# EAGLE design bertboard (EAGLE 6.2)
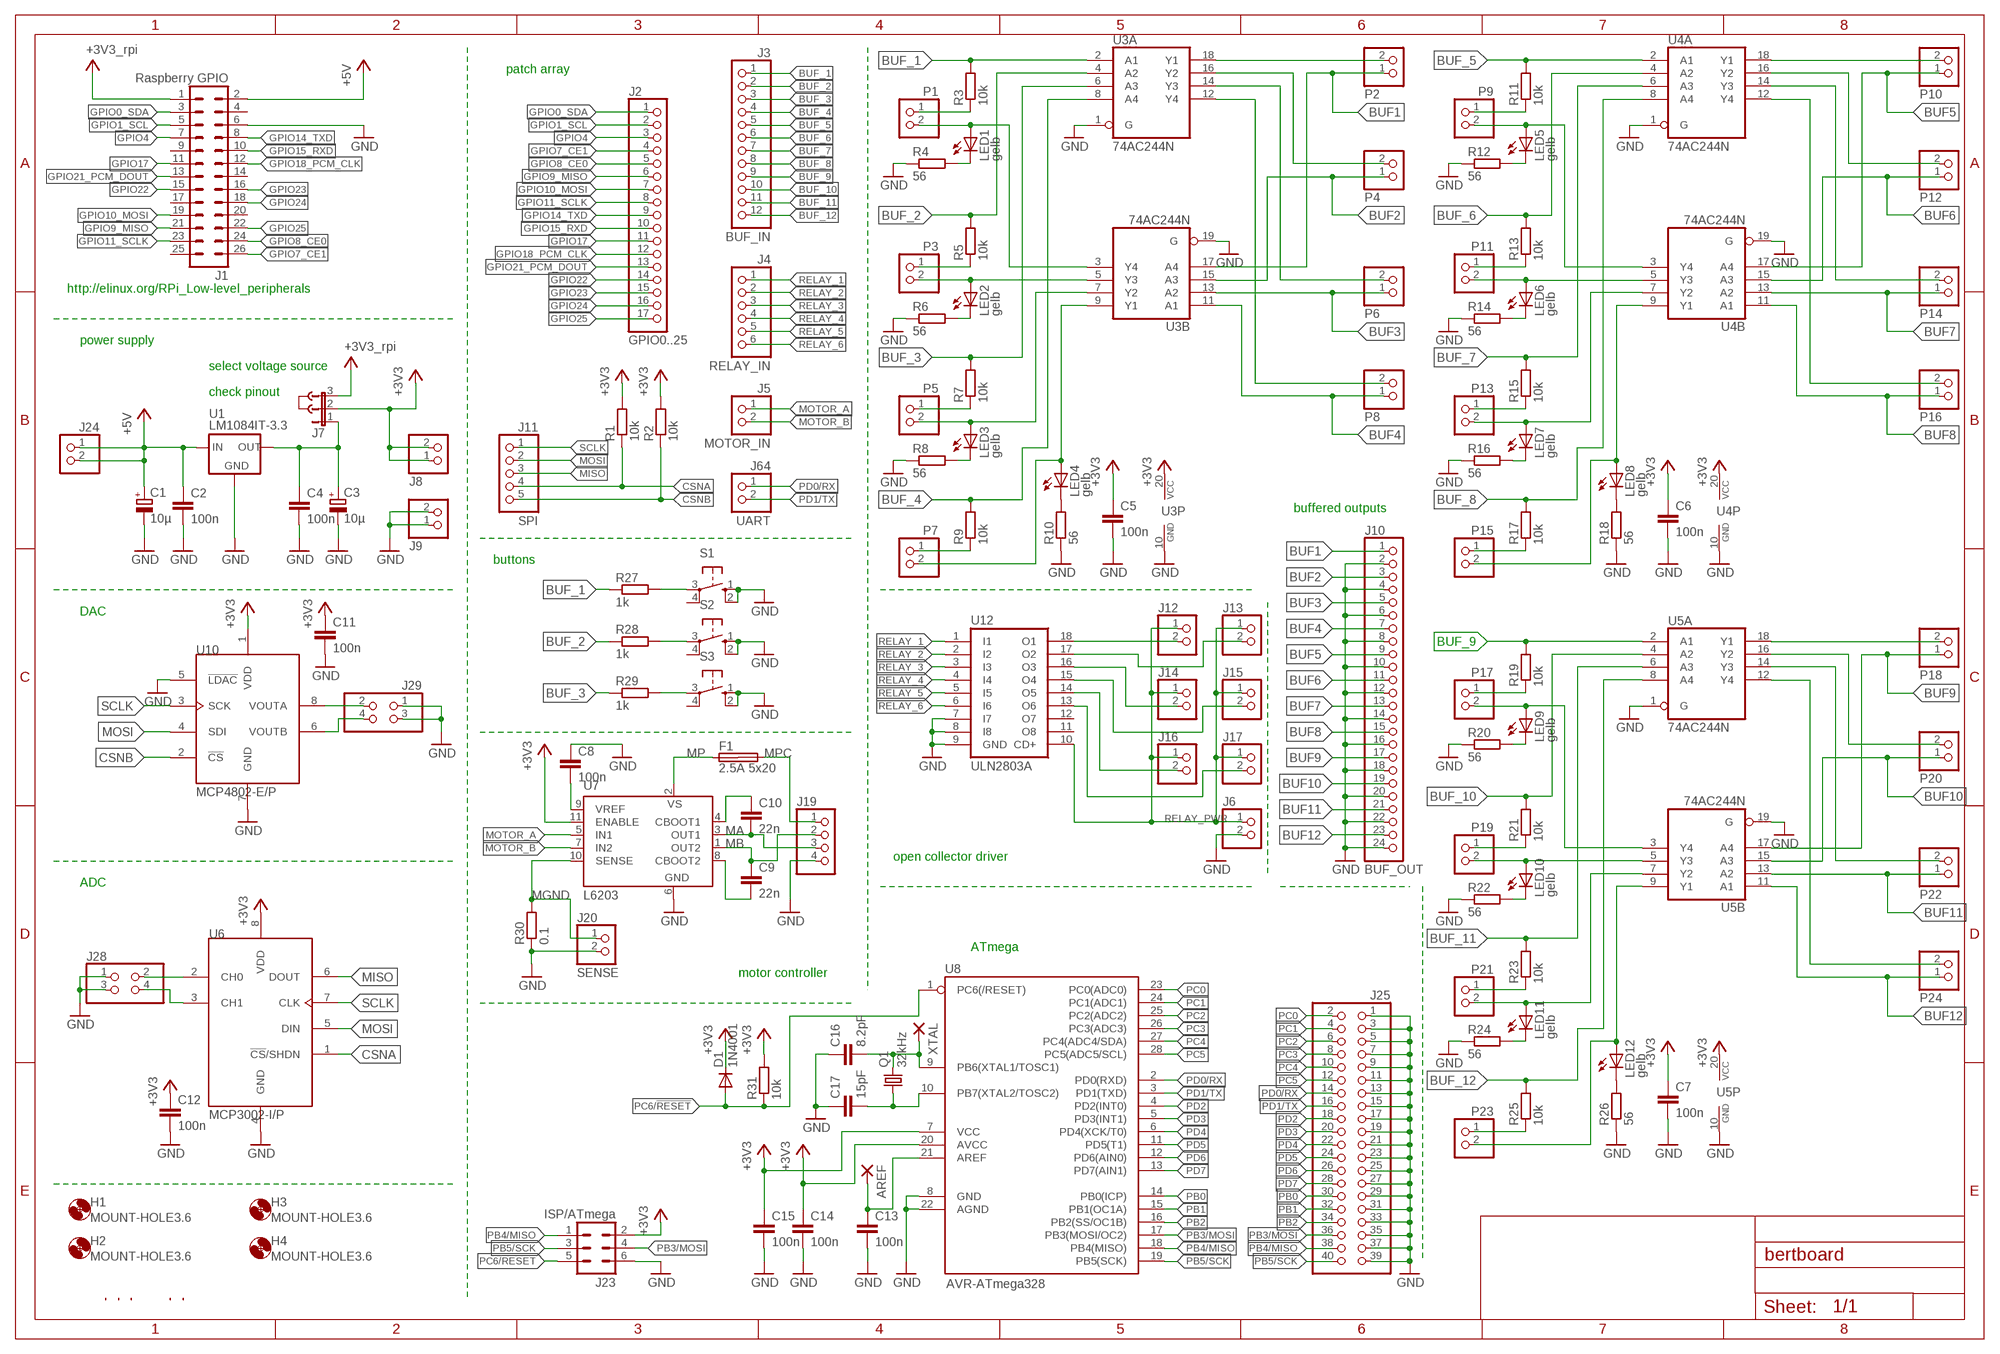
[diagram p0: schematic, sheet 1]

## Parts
AREF  1,6/0,9  [1,6/0,9]
C1  10µ  CPOL-EUE2-5  [E2-5]
C2  100n  C-EUC2012  [C2012]
C3  10µ  CPOL-EUE2-5  [E2-5]
C4  100n  C-EUC2012  [C2012]
C5  100n  C-EUC2012  [C2012]
C6  100n  C-EUC2012  [C2012]
C7  100n  C-EUC2012  [C2012]
C8  100n  C-EUC2012  [C2012]
C9  22n  C-EUC2012  [C2012]
C10  22n  C-EUC2012  [C2012]
C11  100n  C-EUC2012  [C2012]
C12  100n  C-EUC2012  [C2012]
C13  100n  C-EUC2012  [C2012]
C14  100n  C-EUC2012  [C2012]
C15  100n  C-EUC2012  [C2012]
C16  8.2pF  C-EUC2012  [C2012]
C17  15pF  C-EUC2012  [C2012]
D1  1N4001  1N4004  [DO41-10]
F1  2.5A 5x20  SHK20Q  [SHK20Q]
H1  MOUNT-HOLE3.6  [3,6]
H2  MOUNT-HOLE3.6  [3,6]
H3  MOUNT-HOLE3.6  [3,6]
H4  MOUNT-HOLE3.6  [3,6]
J1  Raspberry GPIO  ML26  [ML26]
J2  GPIO0..25  PINHD-1X17  [1X17]
J3  BUF_IN  PINHD-1X12  [1X12]
J4  RELAY_IN  PINHD-1X6  [1X06]
J5  MOTOR_IN  PINHD-1X2  [1X02]
J6  PINHD-1X2  [1X02]
J7  JP2E  [JP2]
J8  PINHD-1X2  [1X02]
J9  PINHD-1X2  [1X02]
J10  BUF_OUT  PINHD-1X24  [1X24]
J11  SPI  PINHD-1X5  [1X05]
J12  PINHD-1X2  [1X02]
J13  PINHD-1X2  [1X02]
J14  PINHD-1X2  [1X02]
J15  PINHD-1X2  [1X02]
J16  PINHD-1X2  [1X02]
J17  PINHD-1X2  [1X02]
J19  PINHD-1X4  [1X04]
J20  SENSE  PINHD-1X2  [1X02]
J23  ISP/ATmega  ML6  [ML6]
J24  PINHD-1X2  [1X02]
J25  PINHD-2X20  [2X20]
J28  PINHD-2X2  [2X02]
J29  PINHD-2X2  [2X02]
J64  UART  PINHD-1X2  [1X02]
J999  JUMPER  [JUMP]
LED1  gelb  LED3MM  [LED3MM]
LED2  gelb  LED3MM  [LED3MM]
LED3  gelb  LED3MM  [LED3MM]
LED4  gelb  LED3MM  [LED3MM]
LED5  gelb  LED3MM  [LED3MM]
LED6  gelb  LED3MM  [LED3MM]
LED7  gelb  LED3MM  [LED3MM]
LED8  gelb  LED3MM  [LED3MM]
LED9  gelb  LED3MM  [LED3MM]
LED10  gelb  LED3MM  [LED3MM]
LED11  gelb  LED3MM  [LED3MM]
LED12  gelb  LED3MM  [LED3MM]
P1  PINHD-1X2  [1X02]
P2  PINHD-1X2  [1X02]
P3  PINHD-1X2  [1X02]
P4  PINHD-1X2  [1X02]
P5  PINHD-1X2  [1X02]
P6  PINHD-1X2  [1X02]
P7  PINHD-1X2  [1X02]
P8  PINHD-1X2  [1X02]
P9  PINHD-1X2  [1X02]
P10  PINHD-1X2  [1X02]
P11  PINHD-1X2  [1X02]
P12  PINHD-1X2  [1X02]
P13  PINHD-1X2  [1X02]
P14  PINHD-1X2  [1X02]
P15  PINHD-1X2  [1X02]
P16  PINHD-1X2  [1X02]
P17  PINHD-1X2  [1X02]
P18  PINHD-1X2  [1X02]
P19  PINHD-1X2  [1X02]
P20  PINHD-1X2  [1X02]
P21  PINHD-1X2  [1X02]
P22  PINHD-1X2  [1X02]
P23  PINHD-1X2  [1X02]
P24  PINHD-1X2  [1X02]
Q1  32kHz  CRYSTALTC26H  [TC26H]
R1  10k  R-EU_M3216  [M3216]
R2  10k  R-EU_M3216  [M3216]
R3  10k  R-EU_M3216  [M3216]
R4  56  R-EU_M3216  [M3216]
R5  10k  R-EU_M3216  [M3216]
R6  56  R-EU_M3216  [M3216]
R7  10k  R-EU_M3216  [M3216]
R8  56  R-EU_M3216  [M3216]
R9  10k  R-EU_M3216  [M3216]
R10  56  R-EU_M3216  [M3216]
R11  10k  R-EU_M3216  [M3216]
R12  56  R-EU_M3216  [M3216]
R13  10k  R-EU_M3216  [M3216]
R14  56  R-EU_M3216  [M3216]
R15  10k  R-EU_M3216  [M3216]
R16  56  R-EU_M3216  [M3216]
R17  10k  R-EU_M3216  [M3216]
R18  56  R-EU_M3216  [M3216]
R19  10k  R-EU_M3216  [M3216]
R20  56  R-EU_M3216  [M3216]
R21  10k  R-EU_M3216  [M3216]
R22  56  R-EU_M3216  [M3216]
R23  10k  R-EU_M3216  [M3216]
R24  56  R-EU_M3216  [M3216]
R25  10k  R-EU_M3216  [M3216]
R26  56  R-EU_M3216  [M3216]
R27  1k  R-EU_M3216  [M3216]
R28  1k  R-EU_M3216  [M3216]
R29  1k  R-EU_M3216  [M3216]
R30  0.1  R-EU_R2512  [R2512]
R31  10k  R-EU_M3216  [M3216]
S1  10-XX  [B3F-10XX]
S2  10-XX  [B3F-10XX]
S3  10-XX  [B3F-10XX]
U1  LM1084IT-3.3  LM1084IT-XX  [LM1084IT-XX]
U3  74AC244N  [DIL20]
U4  74AC244N  [DIL20]
U5  74AC244N  [DIL20]
U6  MCP3002-I/P  [DIL-08]
U7  L6203  [MULTIWATT-11]
U8  AVR-ATmega328  AVR-MEGA8-PPTH  [DIL28-3]
U10  MCP4802-E/P  [DIL-08]
U12  ULN2803A  [DIL18]
U$1  MARKTRIANGLE  [MARK_TRIANGLE]
U$2  MARKTRIANGLE  [MARK_TRIANGLE]
U$3  MARKTRIANGLE  [MARK_TRIANGLE]
U$9  MARKGND  [MARK_GND]
U$19  MARKGND  [MARK_GND]
XTAL  1,6/0,9  [1,6/0,9]

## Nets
+3V3 [Power]: C5.1 C6.1 C7.1 C11.1 C12.1 C14.1 C15.1 D1.C J7.2 J8.1 J8.2 J23.2 R1.2 R2.2 R31.2 U3.20(P:VCC) U4.20(P:VCC) U5.20(P:VCC) U6.8(VDD) U7.11(ENABLE) U8.7(VCC) U8.20(AVCC) U10.1(VDD)
+5V [Power]: C1.+ C2.1 J1.2 J24.1 J24.2 U1.INPUT(IN)
AD0: J28.2 U6.2(CH0)
AD1: J28.4 U6.3(CH1)
BUF1: J10.1 P2.1 U3.17(B:A4)
BUF2: J10.3 P4.1 U3.15(B:A3)
BUF3: J10.5 P6.1 U3.13(B:A2)
BUF4: J10.7 P8.1 U3.11(B:A1)
BUF5: J10.9 P10.1 U4.17(B:A4)
BUF6: J10.11 P12.1 U4.15(B:A3)
BUF7: J10.13 P14.1 U4.13(B:A2)
BUF8: J10.15 P16.1 U4.11(B:A1)
BUF9: J10.17 P18.1 U5.17(B:A4)
BUF10: J10.19 P20.1 U5.15(B:A3)
BUF11: J10.21 P22.1 U5.13(B:A2)
BUF12: J10.23 P24.1 U5.11(B:A1)
BUF_1: J3.1 R3.2 R27.1 U3.2(A:A1)
BUF_2: J3.2 R5.2 R28.1 U3.4(A:A2)
BUF_3: J3.3 R7.2 R29.1 U3.6(A:A3)
BUF_4: J3.4 R9.2 U3.8(A:A4)
BUF_5: J3.5 R11.2 U4.2(A:A1)
BUF_6: J3.6 R13.2 U4.4(A:A2)
BUF_7: J3.7 R15.2 U4.6(A:A3)
BUF_8: J3.8 R17.2 U4.8(A:A4)
BUF_9: J3.9 R19.2 U5.2(A:A1)
BUF_10: J3.10 R21.2 U5.4(A:A2)
BUF_11: J3.11 R23.2 U5.6(A:A3)
BUF_12: J3.12 R25.2 U5.8(A:A4)
CSNA: J11.4 R1.1 U6.1(!CS!/SHDN)
CSNB: J11.5 R2.1 U10.2(!CS)
DA0: J29.2 U10.8(VOUTA)
DA1: J29.4 U10.6(VOUTB)
GND [Power]: C1.- C2.2 C3.- C4.2 C5.2 C6.2 C7.2 C8.1 C11.2 C12.2 C13.2 C14.2 C15.2 C16.1 C17.1 J1.6 J6.2 J9.1 J9.2 J10.2 J10.4 J10.6 J10.8 J10.10 J10.12 J10.14 J10.16 J10.18 J10.20 J10.22 J10.24 J19.4 J20.2 J23.6 J25.1 J25.3 J25.5 J25.7 J25.9 J25.11 J25.13 J25.15 J25.17 J25.19 J25.21 J25.23 J25.25 J25.27 J25.29 J25.31 J25.33 J25.35 J25.37 J25.39 J28.1 J28.3 J29.1 J29.3 R4.1 R6.1 R8.1 R10.1 R12.1 R14.1 R16.1 R18.1 R20.1 R22.1 R24.1 R26.1 R30.1 S1.1(S) S1.2(S1) S2.1(S) S2.2(S1) S3.1(S) S3.2(S1) U1.ADJ_GND(GND) U3.1(A:G) U3.10(P:GND) U3.19(B:G) U4.1(A:G) U4.10(P:GND) U4.19(B:G) U5.1(A:G) U5.10(P:GND) U5.19(B:G) U6.4(GND) U7.6(GND) U8.8(GND) U8.22(AGND) U10.5(!LDAC) U10.7(GND) U12.7(I7) U12.8(I8) U12.9(GND)
GPIO0_SDA: J1.3 J2.1
GPIO1_SCL: J1.5 J2.2
GPIO4: J1.7 J2.3
GPIO7_CE1: J1.26 J2.4
GPIO8_CE0: J1.24 J2.5
GPIO9_MISO: J1.21 J2.6
GPIO10_MOSI: J1.19 J2.7
GPIO11_SCLK: J1.23 J2.8
GPIO14_TXD: J1.8 J2.9
GPIO15_RXD: J1.10 J2.10
GPIO17: J1.11 J2.11
GPIO18_PCM_CLK: J1.12 J2.12
GPIO21_PCM_DOUT: J1.13 J2.13
GPIO22: J1.15 J2.14
GPIO23: J1.16 J2.15
GPIO24: J1.18 J2.16
GPIO25: J1.22 J2.17
J71: C16.2 Q1.2 U8.9(PB6(XTAL1/TOSC1)) XTAL.1(P)
MA [Motor]: C10.2 J19.3 U7.3(OUT1)
MB [Motor]: C9.1 J19.2 U7.1(OUT2)
MGND [Motor]: J20.1 R30.2 U7.10(SENSE)
MISO: J11.3 U6.6(DOUT)
MOSI: J11.2 U6.5(DIN) U10.4(SDI)
MOTOR_A: J5.1 U7.5(IN1)
MOTOR_B: J5.2 U7.7(IN2)
MP [Motor]: F1.1A U7.2(VS)
MPC [Motor]: F1.2A J19.1
N$7 [Power]: C3.+ C4.1 J7.1 U1.OUTPUT(OUT)
N$8: P1.1 R3.1
N$9: LED1.A P1.2 U3.3(B:Y4)
N$10: LED1.K(C) R4.2
N$11: P2.2 U3.18(A:Y1)
N$13: P3.1 R5.1
N$14: P4.2 U3.16(A:Y2)
N$15: LED2.A P3.2 U3.5(B:Y3)
N$16: LED2.K(C) R6.2
N$17: P9.1 R11.1
N$18: P5.1 R7.1
N$19: P6.2 U3.14(A:Y3)
N$20: LED3.K(C) R8.2
N$21: P7.1 R9.1
N$22: LED4.A P7.2 U3.9(B:Y1)
N$23: LED4.K(C) R10.2
N$24: LED3.A P5.2 U3.7(B:Y2)
N$25: LED5.A P9.2 U4.3(B:Y4)
N$26: P8.2 U3.12(A:Y4)
N$27: LED5.K(C) R12.2
N$28: P11.1 R13.1
N$29: LED6.A P11.2 U4.5(B:Y3)
N$30: LED6.K(C) R14.2
N$31: P13.1 R15.1
N$32: P15.1 R17.1
N$33: R27.2 S1.3(P)
N$34: LED8.A P15.2 U4.9(B:Y1)
N$35: LED8.K(C) R18.2
N$36: LED7.A P13.2 U4.7(B:Y2)
N$37: P10.2 U4.18(A:Y1)
N$38: P12.2 U4.16(A:Y2)
N$39: P14.2 U4.14(A:Y3)
N$40: P16.2 U4.12(A:Y4)
N$42: P17.1 R19.1
N$43: LED9.A P17.2 U5.3(B:Y4)
N$44: LED9.K(C) R20.2
N$45: P19.1 R21.1
N$46: LED10.A P19.2 U5.5(B:Y3)
N$47: LED10.K(C) R22.2
N$48: P21.1 R23.1
N$49: LED11.K(C) R24.2
N$50: P23.1 R25.1
N$51: LED12.A P23.2 U5.9(B:Y1)
N$52: LED12.K(C) R26.2
N$53: LED11.A P21.2 U5.7(B:Y2)
N$54: P18.2 U5.18(A:Y1)
N$55: P20.2 U5.16(A:Y2)
N$56: P22.2 U5.14(A:Y3)
N$57: P24.2 U5.12(A:Y4)
N$59: R28.2 S2.3(P)
N$60: R29.2 S3.3(P)
N$62: LED7.K(C) R16.2
N$68: C8.2 U7.9(VREF)
N$72: C10.1 U7.4(CBOOT1)
N$73: C9.2 U7.8(CBOOT2)
N$76: AREF.1(P) C13.1 U8.21(AREF)
N$78: C17.2 Q1.1 U8.10(PB7(XTAL2/TOSC2))
PB0: J25.30 U8.14(PB0(ICP))
PB1: J25.32 U8.15(PB1(OC1A))
PB2: J25.34 U8.16(PB2(SS/OC1B))
PB3/MOSI: J23.4 J25.36 U8.17(PB3(MOSI/OC2))
PB4/MISO: J23.1 J25.38 U8.18(PB4(MISO))
PB5/SCK: J23.3 J25.40 U8.19(PB5(SCK))
PC0: J25.2 U8.23(PC0(ADC0))
PC1: J25.4 U8.24(PC1(ADC1))
PC2: J25.6 U8.25(PC2(ADC2))
PC3: J25.8 U8.26(PC3(ADC3))
PC4: J25.10 U8.27(PC4(ADC4/SDA))
PC5: J25.12 U8.28(PC5(ADC5/SCL))
PC6/!RESET!: D1.A J23.5 R31.1 U8.1(PC6(/RESET))
PD0/RX: J25.14 J64.1 U8.2(PD0(RXD))
PD1/TX: J25.16 J64.2 U8.3(PD1(TXD))
PD2: J25.18 U8.4(PD2(INT0))
PD3: J25.20 U8.5(PD3(INT1))
PD4: J25.22 U8.6(PD4(XCK/T0))
PD5: J25.24 U8.11(PD5(T1))
PD6: J25.26 U8.12(PD6(AIN0))
PD7: J25.28 U8.13(PD7(AIN1))
RELAY_1: J4.1 U12.1(I1)
RELAY_2: J4.2 U12.2(I2)
RELAY_3: J4.3 U12.3(I3)
RELAY_4: J4.4 U12.4(I4)
RELAY_5: J4.5 U12.5(I5)
RELAY_6: J4.6 U12.6(I6)
RELAY_PWR: J6.1 J12.1 J13.1 J14.1 J15.1 J16.1 J17.1 U12.10(CD+)
RLY1: J12.2 U12.18(O1)
RLY2: J13.2 U12.17(O2)
RLY3: J14.2 U12.16(O3)
RLY4: J15.2 U12.15(O4)
RLY5: J16.2 U12.14(O5)
RLY6: J17.2 U12.13(O6)
SCLK: J11.1 U6.7(CLK) U10.3(SCK)
V+ [Power]: J1.1 J7.3 ; supply symbol labelled +3V3_rpi
Unconnected: F1.1B F1.2B J1.4 J1.9 J1.14 J1.17 J1.20 J1.25 S1.4(P1) S2.4(P1) S3.4(P1) U12.11(O8) U12.12(O7)

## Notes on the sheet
- patch array
- http://elinux.org/RPi_Low-level_peripherals
- power supply
- select voltage source
- check pinout
- buffered outputs
- buttons
- DAC
- open collector driver
- ADC
- ATmega
- motor controller

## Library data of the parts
AREF XTAL = wirepad:1,6/0,9: THROUGH-HOLE PAD; PARTNO: n.a.
C1 C3 = rcl:CPOL-EU: POLARIZED CAPACITOR, European symbol; PARTNO: RAD 10/350
C2 C4-C8 C11-C15 = rcl:C-EU: CAPACITOR, European symbol; PARTNO: X7R-G0805 100N
C9 C10 = rcl:C-EU: CAPACITOR, European symbol; PARTNO: X7R-G0805 22N
C16 = rcl:C-EU: CAPACITOR, European symbol; PARTNO: NPO-G0805 8,2P
C17 = rcl:C-EU: CAPACITOR, European symbol; PARTNO: NPO-G0805 15P
D1 = diode:1N4004: DIODE; PARTNO: 1N 4001
F1 = fuse:SHK20Q: FUSE HOLDER 5 x 20 mm, SH contact, E1207 Buerklin 64G6061; OC_FARNELL: unknown; OC_NEWARK: unknown
H1-H4 = holes:MOUNT-HOLE: MOUNTING HOLE with drill center marker; PARTNO: n.a.
J1 = con-ml:ML26: HARTING; OC_FARNELL: unknown; OC_NEWARK: unknown; PARTNO: WSL 26G
J2 = bertboard:PINHD-1X17: PIN HEADER
J3 = bertboard:PINHD-1X12: PIN HEADER; PARTNO: MPE 087-1-012
J4 = pinhead:PINHD-1X6: PIN HEADER; PARTNO: MPE 087-1-006
J5 J6 J8 J9 J12-J17 J20 J24 J64 P1-P9 P11 P13 P15 P17-P24 = pinhead:PINHD-1X2: PIN HEADER; PARTNO: MPE 087-1-002
J7 = jumper:JP2E: JUMPER; PARTNO: MPE 087-1-003
J10 = pinhead:PINHD-1X24: PIN HEADER; PARTNO: MPE 087-1-024
J11 = bertboard:PINHD-1X5: PIN HEADER; PARTNO: MPE 087-1-005
J19 = pinhead:PINHD-1X4: PIN HEADER; PARTNO: MPE 087-1-004
J23 = con-ml:ML6: HARTING; OC_FARNELL: unknown; OC_NEWARK: unknown; PARTNO: WSL 6G
J25 = pinhead:PINHD-2X20: PIN HEADER; PARTNO: MPE 087-2-040
J28 J29 = pinhead:PINHD-2X2: PIN HEADER; PARTNO: MPE 087-2-004
J999 = jumper:JUMPER: JUMPER header; PARTNO: JUMPER 2,54 RT
LED1-LED12 = led:LED: LED; PARTNO: LED 3MM GE
P10 P12 P14 P16 = bertboard:PINHD-1X2: PIN HEADER; PARTNO: MPE 087-1-002
Q1 = crystal:CRYSTAL: CRYSTAL; OC_FARNELL: unknown; OC_NEWARK: unknown; PARTNO: 0,032768
R1-R3 R5 R7 R9 R11 R13 R15 R17 R19 R21 R23 R25 R31 = rcl:R-EU_: RESISTOR, European symbol; PARTNO: SMD 1/4W 10K
R4 R6 R8 R10 R12 R14 R16 R18 R20 R22 R24 R26 = rcl:R-EU_: RESISTOR, European symbol; PARTNO: SMD 1/4W 120
R27-R29 = rcl:R-EU_: RESISTOR, European symbol; PARTNO: SMD 1/4W 1,0K
R30 = rcl:R-EU_: RESISTOR, European symbol; PARTNO: CRA2512 R100E
S1-S3 = switch-omron:10-XX: OMRON SWITCH; MPN: B3F-1000; OC_FARNELL: 176432; OC_NEWARK: 36M3542; PARTNO: TASTER 9302
U1 = bertboard:LM1084IT-XX: VOLTAGE REGULATOR; PARTNO: LM 1084 IT3,3
U3-U5 = 74xx-eu:74*244: Octal BUFFER and LINE DRIVER, 3-state; PARTNO: 74HC 244
U6 = bertboard:MCP3002-I: 2.7V Dual Channel 10-Bit A/D Converter with SPI Serial Interface; PARTNO: Farnell: 1852015
U7 = st-microelectronics:L6203: DMOS FULL BRIDGE DRIVER; MPN: L6203; OC_FARNELL: 1467715; OC_NEWARK: 56P8434; PARTNO: L 6203
U8 = SparkFun:AVR-MEGA8-P: MICROCONTROLLER 8 Kbytes FLASH 1 kbytes SRAM 512 bytes EEPROM USART 4-channel 10 bit ADC 2-channel 8 bit ADC; PARTNO: ATMEGA 328P-PU
U10 = bertboard:MCP4802-E: 8-Bit Dual Voltage Output Digital-to-Analog Converter with Internal VREF and SPI Interface; PARTNO: MCP 4802-E/P
U12 = uln-udn:ULN2803A: DRIVER ARRAY; PARTNO: ULN 2803A
U$1-U$3 U$9 U$19 = bertboard:MARK: mark for e.g. pins; PARTNO: n.a.

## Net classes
1 Power: width 0.5 mm
2 Motor: width 1 mm

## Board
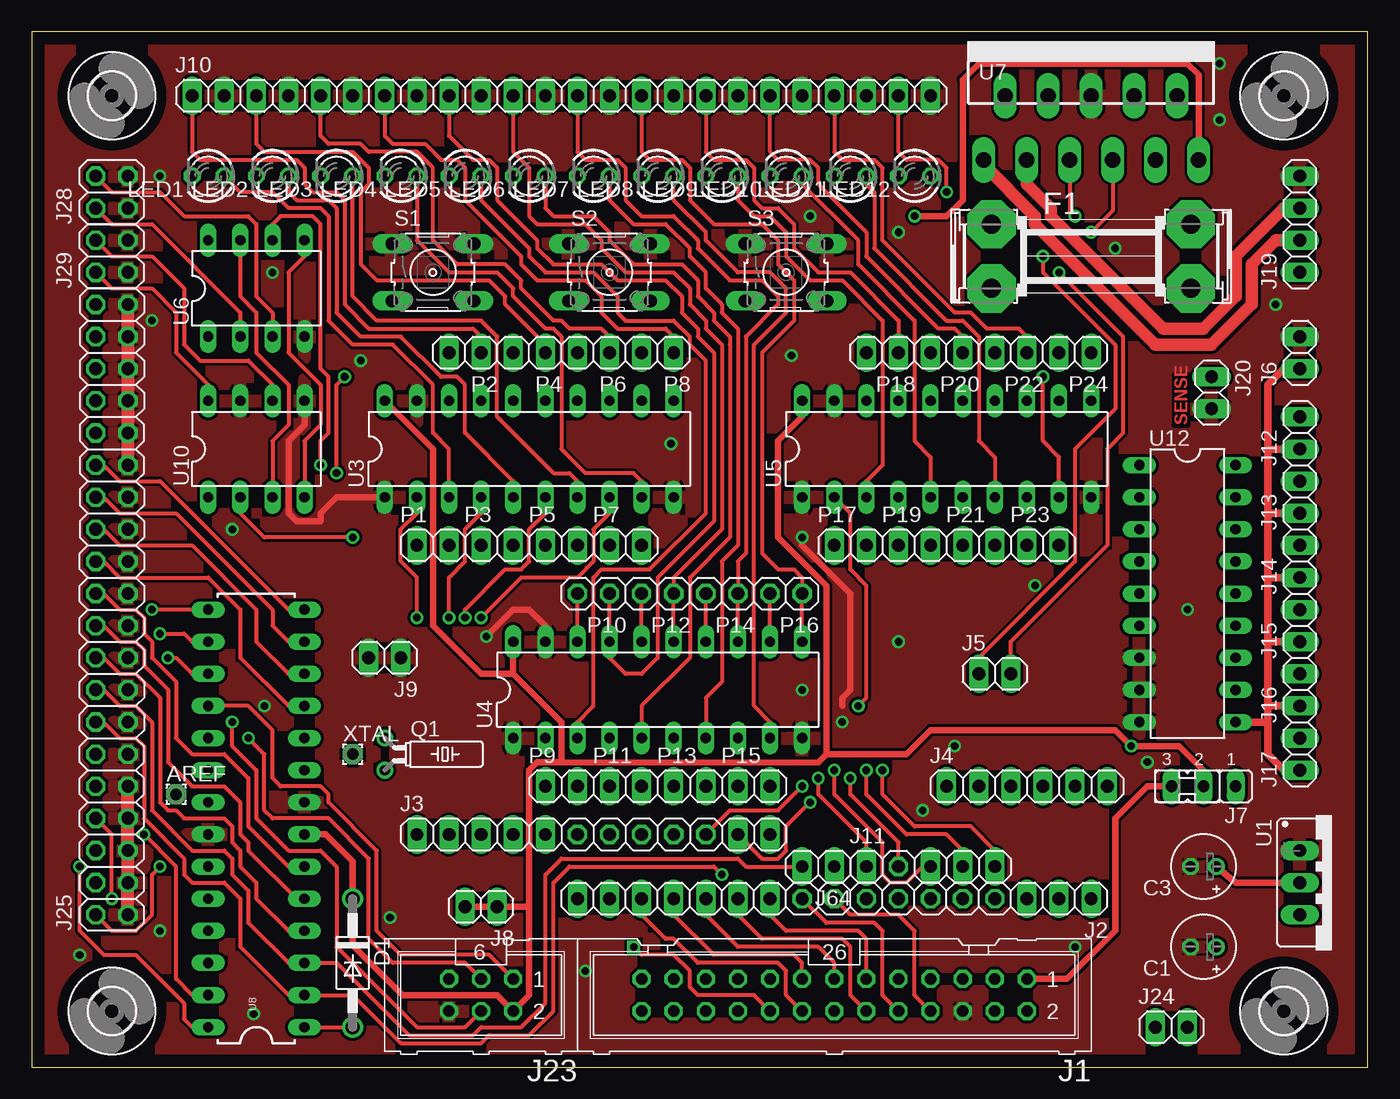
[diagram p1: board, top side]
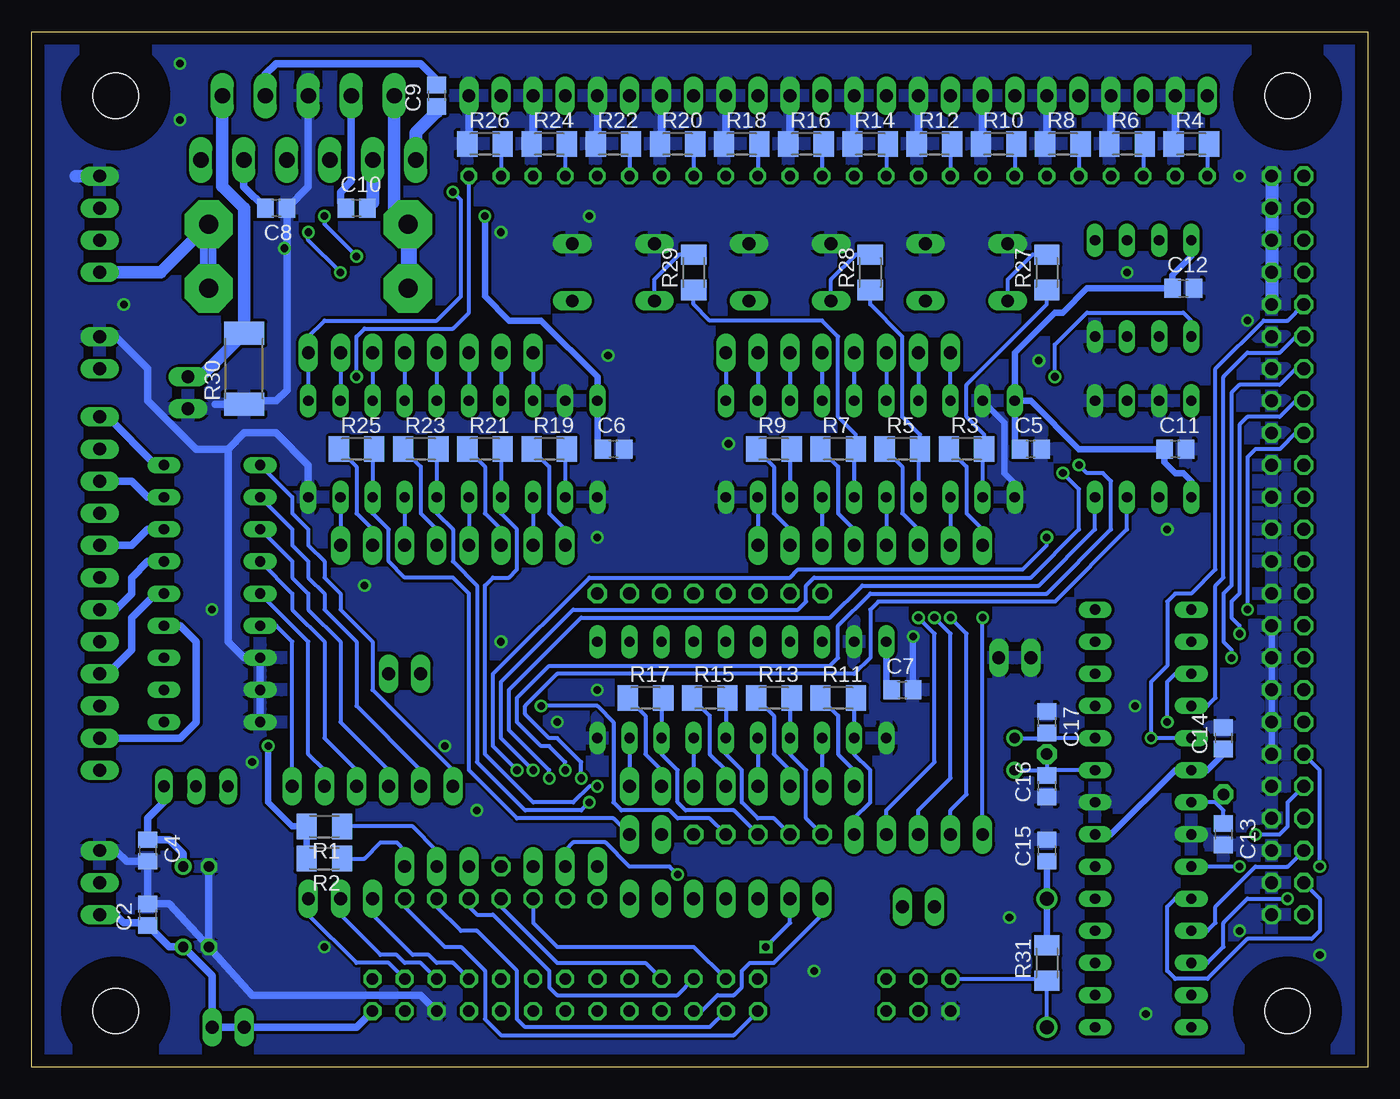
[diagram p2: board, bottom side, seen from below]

Size 105.72 x 81.91 mm. Coordinates in mm from the lower left corner, seen from the top.
Outline: 0,0 105.72,0 105.72,81.91 0,81.91 0,0
Copper layers (1*16): Top 0.035mm / dielectric 1.5mm / Bottom 0.035mm
Design rules: minimum track width 10mil, minimum drill 24mil, track to track 8mil, track to pad 8mil, pad to pad 8mil, via to via 8mil, smd to smd 8mil, copper to edge 40mil, drill to drill 8mil, minimum pad ring 10mil, minimum via ring 8mil, stop-mask expansion 4mil, vias tented up to drill 0mil, thermal gap 10mil

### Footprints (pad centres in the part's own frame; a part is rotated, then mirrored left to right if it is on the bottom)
1,6/0,9 = drill 0.914 pad 1.6 octagon: 1 0,0
E2-5 = drill 0.813 pad 1.27: + -1.016,0 | drill 0.813 pad 1.27 octagon: - 1.016,0
C2012 = smd 1.3 x 1.5: 1 -0.85,0; 2 0.85,0
DO41-10 = drill 1.118: A 5.08,0; C -5.08,0
SHK20Q = drill 1.5 pad 3.81 octagon: 1A -7.874,2.54; 1B -7.874,-2.54; 2A 7.874,2.54; 2B 7.874,-2.54
3,6 = hole 3.6: 0,0
ML26 = drill 0.914 octagon: 1 -15.24,-1.27; 2 -15.24,1.27; 3 -12.7,-1.27; 4 -12.7,1.27; 5 -10.16,-1.27; 6 -10.16,1.27; 7 -7.62,-1.27; 8 -7.62,1.27; 9 -5.08,-1.27; 10 -5.08,1.27; 11 -2.54,-1.27; 12 -2.54,1.27; 13 0,-1.27; 14 0,1.27; 15 2.54,-1.27; 16 2.54,1.27; 17 5.08,-1.27; 18 5.08,1.27; 19 7.62,-1.27; 20 7.62,1.27; 21 10.16,-1.27; 22 10.16,1.27; 23 12.7,-1.27; 24 12.7,1.27; 25 15.24,-1.27; 26 15.24,1.27
1X17 = drill 1.016 long: 1 -20.32,0; 2 -17.78,0; 3 -15.24,0; 11 5.08,0; 12 7.62,0; 13 10.16,0; 14 12.7,0; 15 15.24,0; 16 17.78,0; 17 20.32,0 | drill 1.016 octagon: 4 -12.7,0; 5 -10.16,0; 6 -7.62,0; 7 -5.08,0; 8 -2.54,0; 9 0,0; 10 2.54,0
1X12 = drill 1.016 long: 1 -13.97,0; 2 -11.43,0; 3 -8.89,0; 4 -6.35,0; 5 -3.81,0; 11 11.43,0; 12 13.97,0 | drill 1.016 octagon: 6 -1.27,0; 7 1.27,0; 8 3.81,0; 9 6.35,0; 10 8.89,0
1X06 = drill 1.016 long: 1 -6.35,0; 2 -3.81,0; 3 -1.27,0; 4 1.27,0; 5 3.81,0; 6 6.35,0
1X02 = drill 1.016 long: 1 -1.27,0; 2 1.27,0
JP2 = drill 0.914 long: 1 -2.54,0; 2 0,0; 3 2.54,0
1X24 = drill 1.016 long: 1 -29.21,0; 2 -26.67,0; 3 -24.13,0; 4 -21.59,0; 5 -19.05,0; 6 -16.51,0; 7 -13.97,0; 8 -11.43,0; 9 -8.89,0; 10 -6.35,0; 11 -3.81,0; 12 -1.27,0; 13 1.27,0; 14 3.81,0; 15 6.35,0; 16 8.89,0; 17 11.43,0; 18 13.97,0; 19 16.51,0; 20 19.05,0; 21 21.59,0; 22 24.13,0; 23 26.67,0; 24 29.21,0
1X05 = drill 1.016 long: 1 -5.08,0; 3 0,0; 4 2.54,0; 5 5.08,0 | drill 1.016 octagon: 2 -2.54,0
1X04 = drill 1.016 long: 1 -3.81,0; 2 -1.27,0; 3 1.27,0; 4 3.81,0
ML6 = drill 0.914 octagon: 1 -2.54,-1.27; 2 -2.54,1.27; 3 0,-1.27; 4 0,1.27; 5 2.54,-1.27; 6 2.54,1.27
2X20 = drill 1.016 octagon: 1 -24.13,-1.27; 2 -24.13,1.27; 3 -21.59,-1.27; 4 -21.59,1.27; 5 -19.05,-1.27; 6 -19.05,1.27; 7 -16.51,-1.27; 8 -16.51,1.27; 9 -13.97,-1.27; 10 -13.97,1.27; 11 -11.43,-1.27; 12 -11.43,1.27; 13 -8.89,-1.27; 14 -8.89,1.27; 15 -6.35,-1.27; 16 -6.35,1.27; 17 -3.81,-1.27; 18 -3.81,1.27; 19 -1.27,-1.27; 20 -1.27,1.27; 21 1.27,-1.27; 22 1.27,1.27; 23 3.81,-1.27; 24 3.81,1.27; 25 6.35,-1.27; 26 6.35,1.27; 27 8.89,-1.27; 28 8.89,1.27; 29 11.43,-1.27; 30 11.43,1.27; 31 13.97,-1.27; 32 13.97,1.27; 33 16.51,-1.27; 34 16.51,1.27; 35 19.05,-1.27; 36 19.05,1.27; 37 21.59,-1.27; 38 21.59,1.27; 39 24.13,-1.27; 40 24.13,1.27
2X02 = drill 1.016 octagon: 1 -1.27,-1.27; 2 -1.27,1.27; 3 1.27,-1.27; 4 1.27,1.27
LED3MM = drill 0.813 octagon: A -1.27,0; K 1.27,0
1X02' = drill 1.016 octagon: 1 -1.27,0; 2 1.27,0
TC26H = drill 0.813: 1 -1.27,0; 2 1.27,0
M3216 = smd 1.6 x 2: 1 -1.4,0; 2 1.4,0
R2512 = smd 1.8 x 3.2: 1 -2.8,0; 2 2.8,0
B3F-10XX = drill 1.016 long: 1 -3.251,2.261; 2 3.251,2.261; 3 -3.251,-2.261; 4 3.251,-2.261
LM1084IT-XX = drill 1.016 long: ADJ_GND -2.54,-2.54; INPUT 2.54,-2.54; OUTPUT 0,-2.54
DIL20 = drill 0.813 long: 1 -11.43,-3.81; 2 -8.89,-3.81; 3 -6.35,-3.81; 4 -3.81,-3.81; 5 -1.27,-3.81; 6 1.27,-3.81; 7 3.81,-3.81; 8 6.35,-3.81; 9 8.89,-3.81; 10 11.43,-3.81; 11 11.43,3.81; 12 8.89,3.81; 13 6.35,3.81; 14 3.81,3.81; 15 1.27,3.81; 16 -1.27,3.81; 17 -3.81,3.81; 18 -6.35,3.81; 19 -8.89,3.81; 20 -11.43,3.81
DIL-08 = drill 0.813 long: 1 -3.81,-3.81; 2 -1.27,-3.81; 3 1.27,-3.81; 4 3.81,-3.81; 5 3.81,3.81; 6 1.27,3.81; 7 -1.27,3.81; 8 -3.81,3.81
MULTIWATT-11 = drill 1.2 long: 1 -8.5,-6.35; 2 -6.8,-1.27; 3 -5.1,-6.35; 4 -3.4,-1.27; 5 -1.7,-6.35; 6 0,-1.27; 7 1.7,-6.35; 8 3.4,-1.27; 9 5.1,-6.35; 10 6.8,-1.27; 11 8.5,-6.35
DIL28-3 = drill 0.813 long: 1 -16.51,-3.81; 2 -13.97,-3.81; 3 -11.43,-3.81; 4 -8.89,-3.81; 5 -6.35,-3.81; 6 -3.81,-3.81; 7 -1.27,-3.81; 8 1.27,-3.81; 9 3.81,-3.81; 10 6.35,-3.81; 11 8.89,-3.81; 12 11.43,-3.81; 13 13.97,-3.81; 14 16.51,-3.81; 15 16.51,3.81; 16 13.97,3.81; 17 11.43,3.81; 18 8.89,3.81; 19 6.35,3.81; 20 3.81,3.81; 21 1.27,3.81; 22 -1.27,3.81; 23 -3.81,3.81; 24 -6.35,3.81; 25 -8.89,3.81; 26 -11.43,3.81; 27 -13.97,3.81; 28 -16.51,3.81
DIL18 = drill 0.813 long: 1 -10.16,-3.81; 2 -7.62,-3.81; 3 -5.08,-3.81; 4 -2.54,-3.81; 5 0,-3.81; 6 2.54,-3.81; 7 5.08,-3.81; 8 7.62,-3.81; 9 10.16,-3.81; 10 10.16,3.81; 11 7.62,3.81; 12 5.08,3.81; 13 2.54,3.81; 14 0,3.81; 15 -2.54,3.81; 16 -5.08,3.81; 17 -7.62,3.81; 18 -10.16,3.81

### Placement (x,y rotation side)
AREF  11.43,21.59 0 top
C1  92.71,9.53 180 top
C2  96.52,12.06 90 bottom
C3  92.71,15.88 180 top
C4  96.52,17.15 270 bottom
C5  26.67,48.89 0 bottom
C6  59.69,48.89 0 bottom
C7  36.83,29.85 0 bottom
C8  86.36,67.95 180 bottom
C9  73.66,76.84 90 bottom
C10  80.01,67.95 0 bottom
C11  15.24,48.89 0 bottom
C12  14.61,61.59 0 bottom
C13  11.43,18.42 270 bottom
C14  11.43,26.04 90 bottom
C15  25.4,17.15 90 bottom
C16  25.4,22.23 90 bottom
C17  25.4,27.31 270 bottom
D1  25.4,8.26 270 top
F1  83.82,64.14 0 top
H1  6.35,4.45 0 top
H2  99.06,4.45 0 top
H3  6.35,76.84 0 top
H4  99.06,76.84 0 top
J1  63.5,5.71 180 top
J2  63.5,13.33 180 top
J3  44.45,18.42 0 top
J4  78.74,22.23 0 top
J5  76.2,31.12 0 top
J6  100.33,56.52 90 top
J7  92.71,22.23 180 top
J8  35.56,12.7 180 top
J9  27.94,32.38 180 top
J10  41.91,76.84 0 top
J11  71.12,15.88 0 top
J12  100.33,50.16 90 top
J13  100.33,45.09 90 top
J14  100.33,40 90 top
J15  100.33,34.92 90 top
J16  100.33,29.85 90 top
J17  100.33,24.77 90 top
J19  100.33,66.68 90 top
J20  93.35,53.34 270 top
J23  35.56,5.71 180 top
J24  90.17,3.17 0 top
J25  6.35,36.2 90 top
J28  6.35,69.22 90 top
J29  6.35,64.14 90 top
J64  62.23,15.88 180 top
J999  91.44,22.23 90 top
LED1  13.97,70.48 180 top
LED2  19.05,70.48 180 top
LED3  24.13,70.48 180 top
LED4  29.21,70.48 180 top
LED5  34.29,70.48 180 top
LED6  39.37,70.48 180 top
LED7  44.45,70.48 180 top
LED8  49.53,70.48 180 top
LED9  54.61,70.48 180 top
LED10  59.69,70.48 180 top
LED11  64.77,70.48 180 top
LED12  69.85,70.48 180 top
P1  31.75,41.27 0 top
P2  34.29,56.52 180 top
P3  36.83,41.27 0 top
P4  39.37,56.52 180 top
P5  41.91,41.27 0 top
P6  44.45,56.52 180 top
P7  46.99,41.27 0 top
P8  49.53,56.52 180 top
P9  41.91,22.23 0 top
P10  [1X02']  44.45,37.46 180 top
P11  46.99,22.23 0 top
P12  [1X02']  49.53,37.46 180 top
P13  52.07,22.23 0 top
P14  [1X02']  54.61,37.46 180 top
P15  57.15,22.23 0 top
P16  [1X02']  59.69,37.46 180 top
P17  64.77,41.27 0 top
P18  67.31,56.52 180 top
P19  69.85,41.27 0 top
P20  72.39,56.52 180 top
P21  74.93,41.27 0 top
P22  77.47,56.52 180 top
P23  80.01,41.27 0 top
P24  82.55,56.52 180 top
Q1  27.94,24.77 270 top
R1  82.55,19.05 180 bottom
R2  82.55,16.51 180 bottom
R3  31.75,48.89 0 bottom
R4  13.97,73.03 0 bottom
R5  36.83,48.89 0 bottom
R6  19.05,73.03 0 bottom
R7  41.91,48.89 0 bottom
R8  24.13,73.03 0 bottom
R9  46.99,48.89 0 bottom
R10  29.21,73.03 0 bottom
R11  41.91,29.21 0 bottom
R12  34.29,73.03 0 bottom
R13  46.99,29.21 0 bottom
R14  39.37,73.03 0 bottom
R15  52.07,29.21 0 bottom
R16  44.45,73.03 0 bottom
R17  57.15,29.21 0 bottom
R18  49.53,73.03 0 bottom
R19  64.77,48.89 0 bottom
R20  54.61,73.03 0 bottom
R21  69.85,48.89 0 bottom
R22  59.69,73.03 0 bottom
R23  74.93,48.89 0 bottom
R24  64.77,73.03 0 bottom
R25  80.01,48.89 0 bottom
R26  69.85,73.03 0 bottom
R27  25.4,62.86 90 bottom
R28  39.37,62.86 90 bottom
R29  53.34,62.86 90 bottom
R30  88.9,55.24 90 bottom
R31  25.4,8.26 90 bottom
S1  31.75,62.86 0 top
S2  45.72,62.86 0 top
S3  59.69,62.86 0 top
U1  102.87,14.61 270 top
U3  39.37,48.89 0 top
U4  49.53,29.85 0 top
U5  72.39,48.89 0 top
U6  17.78,61.59 0 top
U7  83.82,78.11 0 top
U8  17.78,19.69 90 top
U10  17.78,48.89 0 top
U12  91.44,37.46 270 top
U$1  86.36,13.33 270 top
U$2  38.1,8.89 0 top
U$3  78.74,8.89 0 top
U$4  MARKGND  [MARK_GND]  103.51,57.78 0 top
U$5  MARKGND  [MARK_GND]  103.2,70.48 0 top
U$6  MARKGND  [MARK_GND]  55.88,79.38 0 top
U$7  MARKGND  [MARK_GND]  66.04,79.38 0 top
U$8  MARKGND  [MARK_GND]  60.96,79.38 0 top
U$9  71.12,79.38 0 top
U$10  MARKGND  [MARK_GND]  50.8,79.38 0 top
U$11  MARKGND  [MARK_GND]  45.72,79.38 0 top
U$12  MARKGND  [MARK_GND]  40.64,79.38 0 top
U$13  MARKGND  [MARK_GND]  35.56,79.38 0 top
U$14  MARKGND  [MARK_GND]  30.48,79.38 0 top
U$15  MARKGND  [MARK_GND]  25.4,79.38 0 top
U$16  MARKGND  [MARK_GND]  20.32,79.38 0 top
U$17  MARKGND  [MARK_GND]  15.24,79.38 0 top
U$18  MARKGND  [MARK_GND]  8.89,72.39 0 top
U$19  8.89,9.53 0 top
XTAL  25.4,24.77 0 top

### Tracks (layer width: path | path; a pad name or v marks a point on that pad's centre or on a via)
+3V3  (via drill 0.6 pad 0.61)
  Top 0.48: 41.91,24.13 62.23,24.13
  Top 0.5: J7.2 92.71,23.5 90.81,25.4 v87,25.4 85.73,26.67 71.12,26.67 69.22,24.77 62.87,24.77 | 62.87,24.77 62.87,38.1 59.05,41.91 59.05,49.53 60.96,51.43 U5.20 | U7.11 92.32,78.5 91.44,79.38 74.93,79.38 73.66,78.11 73.66,68.58 72.39,67.31 v69.85,67.31 | 38.1,31.12 41.91,27.31 41.91,24.13 40.01,24.13 39.37,23.5 39.37,12.7 | U3.20 31.75,48.89 31.75,34.92 35.56,31.12 38.1,31.12 | 38.1,31.12 U4.20 | 39.37,12.7 39.37,5.71 J23.2 36.83,5.71 29.34,5.71 R31.2 D1.C C15.1 23.28,18.42 U8.7 | 62.23,24.13 62.87,24.77 | 39.37,12.7 J8.1 J8.2
  Bottom 0.5: v69.85,67.31 69.85,60.96 67.95,59.05 65.41,59.05 60.96,54.61 U5.20 60.96,49.31 C6.1 | C5.1 27.94,49.31 U3.20 | R31.2 D1.C C15.1 | U8.7 20.32,18.42 15.24,23.5 U8.20 12.7,23.5 11.43,24.77 C14.1 | C7.1 38.1,30.27 U4.20 | U6.8 13.97,64.14 15.45,62.65 C12.1 22.22,61.59 24.13,59.69 24.77,59.69 27.94,56.52 U3.20 | U10.1 13.97,46.35 14.61,46.99 15.24,46.99 16.09,47.84 C11.1 22.86,48.89 26.67,52.7 U3.20 | R2.2 R1.2 85.09,19.05 87,20.96 v87,25.4
+5V
  Bottom 0.61: J1.2 80.01,3.17 J24.1 J24.2 91.44,7.24 C1.+ 94.83,9.53 C2.1 96.73,11.43 98.43,11.43 99.06,12.06 U1.INPUT
AD0
  Top 0.305: J28.2 6.35,66.68 9.53,66.68 16.51,59.69 U6.2
AD1
  Top 0.305: J28.4 6.35,69.22 10.16,69.22 12.07,67.31 17.14,67.31 17.78,66.68 17.78,60.96 19.05,59.69 U6.3
BUF1
  Top 0.305: J10.1 12.7,72.39 13.34,71.76 20.95,71.76 21.59,71.12 21.59,69.85 22.22,69.22 24.13,69.22 24.77,68.58 24.77,60.32 26.67,58.42 34.92,58.42 35.56,57.78 P2.1
  Bottom 0.305: P2.1 U3.17
BUF2
  Top 0.305: J10.3 17.78,73.03 18.41,72.39 25.4,72.39 26.67,71.12 26.67,69.85 26.04,69.22 26.04,63.5 27.3,62.23 36.2,62.23 37.46,60.96 37.46,60.32 40.64,57.15 P4.1
  Bottom 0.305: P4.1 U3.15
BUF3
  Top 0.305: P6.1 45.72,57.78 45.09,58.42 42.55,58.42 41.91,59.05 41.27,59.05 38.73,61.59 38.73,62.23 37.46,63.5 33.66,63.5 31.75,65.41 31.75,71.12 30.48,72.39 26.67,72.39 26.04,73.03 23.49,73.03 22.86,73.66 J10.5
  Bottom 0.305: P6.1 U3.13
BUF4
  Top 0.305: J10.7 27.94,73.66 28.57,73.03 31.11,73.03 32.38,71.76 33.66,71.76 34.29,71.12 34.29,68.58 38.73,64.14 38.73,63.5 40.01,62.23 43.81,62.23 45.09,60.96 45.09,59.69 46.35,58.42 50.16,58.42 50.8,57.78 P8.1
  Bottom 0.305: P8.1 U3.11
BUF5
  Top 0.305: J10.9 33.02,73.66 34.92,71.76 36.2,71.76 36.83,71.12 36.83,68.58 40.01,65.41 40.01,64.77 41.27,63.5 45.09,63.5 46.35,62.23 50.16,62.23 51.44,60.96 51.44,59.69 52.7,58.42 52.7,57.78 53.98,56.52 53.98,43.18 49.53,38.73 49.53,32.38 48.26,31.12 46.99,31.12 45.72,32.38 U4.17 P10.1
BUF6
  Top 0.305: J10.11 38.1,72.39 39.37,71.12 39.37,67.31 40.01,66.68 43.81,66.68 45.09,65.41 45.09,64.77 46.99,62.86 50.8,62.86 52.07,61.59 52.07,60.32 53.34,59.05 53.34,58.42 54.61,57.15 54.61,42.54 50.8,38.73 P12.1 U4.15
BUF7
  Top 0.305: J10.13 43.18,72.39 43.81,71.76 46.35,71.76 46.99,71.12 46.99,68.58 48.26,67.31 50.8,67.31 52.7,65.41 52.7,64.77 55.24,62.23 57.78,62.23 59.05,60.96 59.05,60.32 56.52,57.78 56.52,40.64 55.88,40 P14.1 U4.13
BUF8
  Top 0.305: J10.15 48.26,72.39 48.89,71.76 51.44,71.76 52.07,71.12 52.07,68.58 53.98,66.68 57.78,66.68 59.05,65.41 59.05,63.5 60.32,62.23 60.32,59.05 57.78,56.52 57.78,40.64 59.05,39.37 60.32,39.37 60.96,38.73 P16.1 U4.11
BUF9
  Top 0.305: J10.17 53.34,72.39 53.98,71.76 56.52,71.76 57.15,71.12 57.15,68.58 57.78,67.95 59.05,67.95 60.32,66.68 60.32,64.77 62.23,62.86 64.77,62.86 68.58,59.05 P18.1
  Bottom 0.305: P18.1 U5.17
BUF10
  Top 0.305: P20.1 73.66,57.78 73.03,58.42 71.76,58.42 66.04,64.14 66.04,66.04 62.23,69.85 62.23,71.12 61.59,71.76 59.05,71.76 58.42,72.39 J10.19
  Bottom 0.305: P20.1 U5.15
BUF11
  Top 0.305: J10.21 63.5,72.39 64.14,71.76 66.68,71.76 67.31,71.12 67.31,65.41 73.03,59.69 74.3,59.69 75.57,58.42 78.11,58.42 78.74,57.78 P22.1
  Bottom 0.305: P22.1 U5.13
BUF12  (via drill 0.6 pad 0.6)
  Top 0.305: v72.39,69.22 72.39,71.12 71.76,71.76 69.22,71.76 68.58,72.39 J10.23
  Bottom 0.305: U5.11 P24.1 83.82,57.78 82.55,59.05 73.66,59.05 71.76,60.96 71.76,68.58 v72.39,69.22
BUF_1  (via drill 0.6 pad 0.61)
  Top 0.305: v30.48,35.56 30.48,38.73 29.21,40 29.21,42.54 30.48,43.81 U3.2
  Bottom 0.305: U3.2 30.48,48.77 R3.2 30.35,50.03 31.75,51.43 31.75,53.98 25.4,60.32 R27.1 | J3.1 v30.48,35.56
BUF_2  (via drill 0.6 pad 0.61)
  Top 0.305: v33.02,35.56 33.02,38.73 34.29,40 34.29,42.54 35.56,43.81 U3.4
  Bottom 0.305: U3.4 35.56,48.77 R5.2 35.43,50.03 36.83,51.43 36.83,57.78 39.37,60.32 R28.1 | J3.2 33.02,20.32 31.75,21.59 31.75,34.29 v33.02,35.56
BUF_3  (via drill 0.6 pad 0.61)
  Top 0.305: v34.29,35.56 34.29,36.2 37.46,39.37 38.73,39.37 39.37,40 39.37,42.54 40.64,43.81 U3.6
  Bottom 0.305: U3.6 40.64,48.77 R7.2 40.51,50.03 41.91,51.43 41.91,57.78 43.18,59.05 52.07,59.05 53.34,60.32 R29.1 | J3.3 35.56,20.32 33.02,22.86 33.02,34.29 v34.29,35.56
BUF_4  (via drill 0.6 pad 0.61)
  Top 0.305: U3.8 45.72,43.81 44.45,42.54 44.45,40 43.18,38.73 38.73,38.73 v35.56,35.56
  Bottom 0.305: R9.2 45.72,48.77 U3.8 | J3.4 38.1,20.32 34.29,24.13 34.29,34.29 v35.56,35.56
BUF_5
  Bottom 0.305: R11.2 40.64,29.08 U4.2 40.64,24.77 39.37,23.5 39.37,20.96 40.64,19.69 J3.5
BUF_6
  Bottom 0.305: R13.2 45.72,29.08 U4.4 45.72,24.77 44.45,23.5 44.45,19.69 J3.6
BUF_7
  Bottom 0.305: R15.2 50.8,29.08 U4.6 50.8,24.77 49.53,23.5 49.53,20.96 48.26,19.69 46.99,19.69 J3.7
BUF_8
  Bottom 0.305: R17.2 55.88,29.21 U4.8 55.88,24.77 54.61,23.5 54.61,20.96 53.98,20.32 50.16,20.32 J3.8
BUF_9  (via drill 0.6 pad 0.61)
  Top 0.305: v65.41,28.58 66.04,29.21 66.04,38.1 64.77,39.37 64.77,43.81 U5.2
  Bottom 0.305: R19.2 63.5,48.77 U5.2 | J3.9 52.07,19.69 54.61,19.69 55.24,20.32 59.05,20.32 59.69,20.96 59.69,27.31 60.96,28.58 v65.41,28.58
BUF_10  (via drill 0.6 pad 0.61)
  Top 0.305: J3.10 55.24,20.32 59.05,20.32 v60.96,22.23
  Bottom 0.305: R21.2 68.58,48.77 U5.4 68.58,43.81 67.31,42.54 67.31,39.37 67.95,38.73 69.22,38.73 69.85,38.1 69.85,24.77 66.04,20.96 62.87,20.96 61.59,22.23 v60.96,22.23
BUF_11  (via drill 0.6 pad 0.61)
  Top 0.305: J3.11 57.78,16.51 59.05,16.51 59.69,17.15 59.69,19.05 v61.59,20.96
  Bottom 0.305: R23.2 73.66,48.77 U5.6 73.66,43.81 72.39,42.54 72.39,40 70.48,38.1 70.48,24.13 66.68,20.32 62.23,20.32 v61.59,20.96
BUF_12
  Bottom 0.305: R25.2 78.74,48.77 U5.8 78.74,43.81 77.47,42.54 77.47,40 76.2,38.73 72.39,38.73 71.12,37.46 71.12,23.5 67.31,19.69 59.69,19.69 J3.12
CSNA  (via drill 0.6 pad 0.61)
  Top 0.305: J11.4 73.66,17.15 72.39,18.42 69.22,18.42 66.04,21.59 v66.04,23.5 | v24.13,46.99 24.13,53.98 v24.77,54.61
  Bottom 0.305: U6.1 13.97,59.05 14.61,59.69 22.22,59.69 24.77,57.15 v24.77,54.61 | v66.04,23.5 68.58,26.04 68.58,30.48 62.87,36.2 45.09,36.2 44.45,36.83 44.45,38.1 43.81,38.73 26.67,38.73 22.86,42.54 22.86,45.72 v24.13,46.99 | J11.4 73.66,17.15 75.57,19.05 R1.1
CSNB  (via drill 0.6 pad 0.61)
  Top 0.305: v67.31,23.5 67.31,21.59 69.85,19.05 74.3,19.05 76.2,17.15 J11.5 | v25.4,41.91 18.41,41.91 16.51,43.81 U10.2
  Bottom 0.305: v67.31,23.5 69.22,25.4 69.22,31.12 61.59,38.73 45.72,38.73 45.09,39.37 27.3,39.37 25.4,41.27 v25.4,41.91 | R2.1 79.38,16.51 78.11,17.78 76.84,17.78 76.2,17.15 J11.5
DA0
  Top 0.305: J29.2 6.35,61.59 9.53,61.59 11.43,59.69 11.43,56.52 13.97,53.98 U10.8
DA1
  Top 0.305: J29.4 6.35,64.14 9.53,64.14 12.07,61.59 12.07,57.15 13.34,55.88 17.14,55.88 19.05,53.98 U10.6
GND  (via drill 0.6 pad 0.61)
  Top 0.5: U10.5 21.59,50.8 20.32,49.53 20.32,43.81 20.95,43.18 22.86,43.18 22.86,43.81 24.13,45.09 U3.1 | U4.19 40.64,34.92 39.37,36.2 38.1,36.2 v35.98,34.07 | v60.96,41.91 60.96,41.27 64.77,37.46 64.77,29.85 64.14,29.21 64.14,28.58
  Top 1.016: J25.39 J25.37 J25.35 J25.33 J25.31 J25.29 | J25.1 J25.3 J25.5 J25.7 J25.9
  Bottom 0.5: J25.19 J25.17 J25.15 J25.13 J25.11 | 26.04,49.11 C5.2 | C7.2 v35.98,34.07 | U3.19 28.75,50.98 28.75,46.96 27.94,46.15 U3.1
  Bottom 0.61: J1.6 74.93,5.71 88.27,5.71 C1.- | C1.- C3.- | C1.- 94.83,12.91 C2.2 C4.2 98.21,16.3 99.06,17.15 U1.ADJ_GND | U12.9 U12.8 U12.7 88.9,32.38 90.17,33.66 90.17,48.89 | J10.24 71.12,73.03 R26.1 | J10.22 66.04,73.03 R24.1 | J10.20 60.96,73.03 R22.1 | J10.18 55.88,73.03 R20.1 | J10.16 50.8,73.03 R18.1 | J10.14 45.72,73.03 R16.1 | J10.12 40.64,73.03 R14.1 | J10.10 35.56,73.03 R12.1 | J10.8 30.48,73.03 R10.1 | J10.6 25.4,73.03 R8.1 | J10.4 20.32,73.03 R6.1 | J10.2 15.24,73.03 R4.1 | U7.6 83.82,69.64 C8.1 85.51,53.55 86.36,52.7 88.64,52.7 R30.1 91.18,52.45 | J6.2 99.06,57.78 96.52,55.24 96.52,52.7 92.71,48.89 90.17,48.89 | U5.10 83.82,47.62 86.36,50.16 88.9,50.16 90.17,48.89
  Bottom 1: J19.4 102.23,70.48
  Bottom 1.016: J28.3 J28.1 J29.3 J29.1 J25.39
  other vias: 68.58,33.66 79.38,38.1 60.96,29.85 64.14,27.31 17.57,4.23 70.48,20.32 82.55,9.53 73.03,25.4 68.58,66.04 61.59,67.31 91.44,36.2 85.73,64.77 93.98,74.93 93.98,79.38 98.43,60.32 88.27,24.13 43.81,7.62 18.41,28.58 15.88,42.54 10.16,10.79 3.81,8.89 28.36,11.85 50.59,49.31 60.11,56.3 9.53,59.05 10.16,70.48 19.05,62.86 26.04,55.88
  pour Top (isolate 0.229): -0.63,87 -0.63,-6.99 107.32,-6.99 107.32,87
  pour Bottom (isolate 0.229): -7.62,83.82 -7.62,-2.54 108.59,-2.54 108.59,83.82
GPIO0_SDA
  Bottom 0.305: J1.3 77.47,8.26 80.01,8.26 83.82,12.06 J2.1
GPIO1_SCL
  Bottom 0.305: J1.5 74.93,8.26 76.2,8.26 76.84,8.89 78.11,8.89 81.28,12.06 J2.2
GPIO4
  Bottom 0.305: J1.7 72.39,8.26 73.66,8.26 74.3,8.89 75.57,8.89 78.74,12.06 J2.3
GPIO7_CE1
  Bottom 0.305: J2.4 76.2,12.7 73.03,9.53 71.76,9.53 69.85,7.62 69.85,3.81 68.58,2.54 50.16,2.54 J1.26
GPIO8_CE0
  Bottom 0.305: J1.24 52.07,3.17 66.68,3.17 67.31,3.81 67.31,7.62 70.48,10.79 71.76,10.79 73.66,12.7 J2.5
GPIO9_MISO
  Bottom 0.305: J2.6 71.12,12.7 70.48,12.06 69.22,12.06 64.77,7.62 64.77,6.35 64.14,5.71 54.61,5.71 J1.21
GPIO10_MOSI
  Bottom 0.305: J2.7 68.58,12.7 64.14,8.26 57.15,8.26 J1.19
GPIO11_SCLK
  Bottom 0.305: J2.8 66.04,11.43 64.14,9.53 53.34,9.53 J1.23
GPIO14_TXD
  Top 0.305: J1.8 69.85,5.71 69.85,10.79 68.58,12.06 64.77,12.06 J2.9
GPIO15_RXD
  Top 0.305: J1.10 67.31,5.71 67.31,10.79 66.68,11.43 62.87,11.43 J2.10
GPIO17
  Top 0.305: J1.11 66.04,10.16 65.41,10.79 59.69,10.79 58.42,12.06 J2.11
GPIO18_PCM_CLK
  Top 0.305: J1.12 64.77,5.71 64.77,9.53 64.14,10.16 57.78,10.16 55.88,12.06 J2.12
GPIO21_PCM_DOUT
  Top 0.305: J1.13 63.5,8.26 62.23,9.53 55.88,9.53 53.34,12.06 J2.13
GPIO22
  Top 0.305: J1.15 60.96,8.26 60.32,8.89 53.98,8.89 50.8,12.06 J2.14
GPIO23
  Top 0.305: J1.16 59.69,5.71 59.69,7.62 59.05,8.26 52.7,8.26 50.8,10.16 50.16,10.16 48.26,12.06 J2.15
GPIO24  (via drill 0.6)
  Top 0.305: J1.18 57.15,5.71 52.7,5.71 52.07,6.35 52.07,7.62 50.8,8.89 48.26,8.89 v47.62,9.53
  Bottom 0.305: v47.62,9.53 45.72,11.43 J2.16
GPIO25
  Top 0.305: 43.18,12.06 J2.17
  Bottom 0.305: J1.22 52.7,4.45 51.44,5.71 50.16,5.71 49.53,6.35 49.53,7.62 48.89,8.26 46.99,8.26 43.18,12.06 J2.17
J71
  Bottom 0.305: U8.9 24.98,23.5 C16.2 | Q1.2 25.82,23.5 C16.2 | XTAL.1 C16.2
MA
  Top 1: J19.3 99.06,67.95 95.25,64.14 95.25,60.96 92.71,58.42 89.54,58.42 80.65,67.31 80.65,67.95 78.74,69.85 78.74,70.48 78.72,70.48 U7.3
  Bottom 1.016: U7.3 78.72,68.39 C10.2
MB
  Top 1: U7.1 75.32,71.37 79.38,67.31 79.38,66.68 88.9,57.15 93.35,57.15 96.52,60.32 96.52,63.5 98.43,65.41 J19.2
  Bottom 1.016: C9.1 73.66,75.57 75.32,73.91 U7.1
MGND
  Bottom 1: U7.10 90.62,69.67 88.9,67.95 R30.2 92.34,54.61 J20.1
MISO  (via drill 0.6 pad 0.61)
  Top 0.305: J11.3 70.48,15.88 69.22,14.61 67.95,14.61 67.31,15.24 67.31,17.78 63.5,21.59 v63.5,23.5 | v22.86,47.62 22.86,49.53 23.49,50.16 23.49,54.61 22.86,55.24 22.86,66.68 22.22,67.31 19.68,67.31 19.05,66.68 U6.6
  Bottom 0.305: v63.5,23.5 63.5,24.13 64.77,25.4 65.41,25.4 67.31,27.31 67.31,29.21 64.77,31.75 42.55,31.75 41.91,32.38 41.91,34.92 39.37,37.46 25.4,37.46 20.32,42.54 20.32,46.35 20.95,46.99 22.22,46.99 v22.86,47.62
MOSI  (via drill 0.6 pad 0.61)
  Top 0.305: U6.5 21.59,64.14 20.32,62.86 20.32,56.52 22.86,53.98 22.86,50.8 21.59,49.53 U10.4 | J11.2 68.58,17.78 64.77,21.59 v64.77,22.86
  Bottom 0.305: v64.77,22.86 64.77,23.5 67.95,26.67 67.95,29.85 62.23,35.56 42.55,35.56 40.01,38.1 26.04,38.1 21.59,42.54 U10.4
MOTOR_A  (via drill 0.6 pad 0.61)
  Top 0.305: J5.1 74.93,32.38 82.55,40 82.55,48.89 85.73,52.07 85.73,57.15 80.01,62.86 v80.01,64.14 | U7.5 82.12,67.74 v82.55,67.31
  Bottom 0.305: v82.55,67.31 82.55,66.68 v80.01,64.14
MOTOR_B  (via drill 0.6 pad 0.61)
  Top 0.305: J5.2 77.47,33.66 85.09,41.27 85.09,48.89 86.36,50.16 86.36,57.78 v81.28,62.86 | U7.7 85.52,67.74 v83.82,66.04
  Bottom 0.305: v81.28,62.86 83.82,65.41 v83.82,66.04
MP
  Bottom 0.5: 75.57,66.68 F1.1A 76.2,66.68
  Bottom 0.65: 75.57,66.68 75.57,61.59 | 76.2,66.68 76.2,61.59
  Bottom 1: U7.2 77.02,67.75
  Bottom 1.016: 77.02,67.75 F1.1A
MPC
  Bottom 0.5: 91.44,66.68 F1.2A 92.08,66.68
  Bottom 0.65: 91.44,66.68 91.44,61.59 | 92.08,61.59 92.08,66.68
  Bottom 1: J19.1 95.5,62.86 F1.2A
N$7
  Top 0.5: U1.OUTPUT 95.25,14.61 C3.+
  Bottom 0.61: C3.+ 93.73,16.89 94.83,18 C4.1 96.52,19.69 95.25,20.96 J7.1
N$8
  Bottom 0.305: R3.1 31.75,47.49 31.75,43.81 30.48,42.54 P1.1
N$9
  Top 0.305: LED1.A 16.51,69.22 19.05,69.22 20.32,67.95 22.86,67.95 23.49,67.31 23.49,59.05 25.4,57.15 28.57,57.15 31.75,53.98 31.75,50.16 33.02,48.89 U3.3
  Bottom 0.305: U3.3 P1.2
N$10
  Bottom 0.305: R4.2 12.7,72.9 LED1.K
N$11
  Bottom 0.305: U3.18 P2.2
N$13
  Bottom 0.305: R5.1 36.83,47.49 36.83,43.81 35.56,42.54 P3.1
N$14
  Bottom 0.305: P4.2 U3.16
N$15
  Top 0.305: LED2.A 20.32,69.22 20.95,68.58 23.49,68.58 24.13,67.95 24.13,59.69 26.04,57.78 29.21,57.78 32.38,54.61 33.66,54.61 34.29,53.98 34.29,50.16 38.1,46.35 U3.5
  Bottom 0.305: U3.5 P3.2
N$16
  Bottom 0.305: R6.2 17.78,72.9 LED2.K
N$17
  Bottom 0.305: R11.1 41.91,27.81 41.91,24.77 40.64,23.5 P9.1
N$18
  Bottom 0.305: R7.1 41.91,47.49 41.91,43.81 40.64,42.54 P5.1
N$19
  Bottom 0.305: P6.2 U3.14
N$20
  Bottom 0.305: R8.2 22.86,72.9 LED3.K
N$21
  Bottom 0.305: R9.1 46.99,47.49 46.99,43.81 45.72,42.54 P7.1
N$22
  Top 0.305: LED4.A 30.48,65.41 33.02,62.86 36.83,62.86 38.1,61.59 38.1,60.96 40.64,58.42 41.27,58.42 41.91,57.78 41.91,48.89 43.81,46.99 47.62,46.99 48.26,46.35 U3.9
  Bottom 0.305: U3.9 P7.2
N$23
  Bottom 0.305: R10.2 27.94,72.9 LED4.K
N$24
  Top 0.305: U3.7 43.18,46.35 42.55,46.99 41.27,46.99 36.83,51.43 36.83,57.78 35.56,59.05 27.3,59.05 25.4,60.96 LED3.A
  Bottom 0.305: U3.7 P5.2
N$25
  Top 0.305: LED5.A 35.56,68.58 39.37,64.77 39.37,64.14 40.64,62.86 44.45,62.86 46.35,60.96 46.35,59.69 46.99,59.05 50.8,59.05 52.07,57.78 52.07,57.15 53.34,55.88 53.34,43.81 48.89,39.37 45.09,39.37 44.45,38.73 44.45,28.58 43.18,27.31 U4.3
  Bottom 0.305: U4.3 P9.2
N$26
  Bottom 0.305: P8.2 U3.12
N$27
  Bottom 0.305: R12.2 33.02,72.9 LED5.K
N$28
  Bottom 0.305: R13.1 46.99,27.81 46.99,24.77 45.72,23.5 P11.1
N$29
  Top 0.305: LED6.A 40.64,67.95 41.27,67.31 44.45,67.31 45.72,66.04 45.72,65.41 47.62,63.5 51.44,63.5 52.7,62.23 52.7,60.96 53.98,59.69 53.98,59.05 55.24,57.78 55.24,57.15 55.24,41.91 52.07,38.73 52.07,32.38 48.26,28.58 U4.5
  Bottom 0.305: U4.5 P11.2
N$30
  Bottom 0.305: R14.2 38.1,72.9 LED6.K
N$31
  Bottom 0.305: R15.1 52.07,27.81 52.07,24.77 50.8,23.5 P13.1
N$32
  Bottom 0.305: R17.1 57.15,27.81 57.15,24.77 55.88,23.5 P15.1
N$33
  Bottom 0.305: S1.3 28.5,62.31 26.54,64.27 R27.2
N$34
  Top 0.305: U4.9 58.42,27.31 57.15,28.58 57.15,57.15 59.69,59.69 59.69,61.59 58.42,62.86 55.88,62.86 53.34,65.41 53.34,66.04 50.8,68.58 LED8.A
  Bottom 0.305: U4.9 P15.2
N$35
  Bottom 0.305: R18.2 48.26,72.9 LED8.K
N$36
  Top 0.305: U4.7 53.34,29.21 54.61,30.48 54.61,40 55.88,41.27 55.88,58.42 54.61,59.69 54.61,60.32 53.34,61.59 53.34,62.86 52.07,64.14 52.07,64.77 50.16,66.68 47.62,66.68 45.72,68.58 LED7.A
  Bottom 0.305: U4.7 P13.2
N$37
  Top 0.305: U4.18 P10.2
N$38
  Top 0.305: U4.16 P12.2
N$39
  Top 0.305: U4.14 P14.2
N$40
  Top 0.305: U4.12 P16.2
N$42
  Bottom 0.305: R19.1 64.77,47.49 64.77,43.81 63.5,42.54 P17.1
N$43
  Top 0.305: LED9.A 55.88,68.58 57.15,67.31 58.42,67.31 59.69,66.04 59.69,64.14 61.59,62.23 64.14,62.23 67.31,59.05 67.31,47.62 66.04,46.35 U5.3
  Bottom 0.305: U5.3 P17.2
N$44
  Bottom 0.305: R20.2 53.34,72.9 LED9.K
N$45
  Bottom 0.305: R21.1 69.85,47.49 69.85,43.81 68.58,42.54 P19.1
N$46
  Top 0.305: U5.5 71.12,48.26 69.85,49.53 69.85,59.05 65.41,63.5 65.41,65.41 60.96,69.85 LED10.A
  Bottom 0.305: U5.5 P19.2
N$47
  Bottom 0.305: R22.2 58.42,72.9 LED10.K
N$48
  Bottom 0.305: R23.1 74.93,47.49 74.93,43.81 73.66,42.54 P21.1
N$49
  Bottom 0.305: R24.2 63.5,72.9 LED11.K
N$50
  Bottom 0.305: R25.1 80.01,47.49 80.01,43.81 78.74,42.54 P23.1
N$51  (via drill 0.6 pad 0.61)
  Top 0.305: U5.9 81.28,48.26 80.01,49.53 v80.01,54.61
  Bottom 0.305: U5.9 P23.2 | v80.01,54.61 80.01,57.78 79.38,58.42 72.39,58.42 71.12,59.69 LED12.A
N$52
  Bottom 0.305: R26.2 68.58,72.9 LED12.K
N$53
  Top 0.305: U5.7 76.2,48.26 74.93,49.53 74.93,57.78 73.66,59.05 72.39,59.05 66.68,64.77 66.68,69.22 66.04,69.85 LED11.A
  Bottom 0.305: U5.7 P21.2
N$54
  Bottom 0.305: P18.2 U5.18
N$55
  Bottom 0.305: P20.2 U5.16
N$56
  Bottom 0.305: P22.2 U5.14
N$57
  Bottom 0.305: P24.2 U5.12
N$59
  Bottom 0.305: S2.3 42.47,62.31 40.51,64.27 R28.2
N$60
  Bottom 0.305: S3.3 56.44,62.31 54.48,64.27 R29.2
N$62
  Bottom 0.305: R16.2 43.18,72.9 LED7.K
N$68
  Bottom 0.61: C8.2 88.92,69.66 U7.9
N$72
  Bottom 0.61: U7.4 80.42,70.08 81.28,69.22 81.28,68.37 C10.1
N$73
  Bottom 0.61: U7.8 87.22,78.52 86.36,79.38 74.93,79.38 73.66,78.11 C9.2
N$76
  Bottom 0.305: C13.1 11.43,20.32 12.07,20.96 | 12.07,20.96 U8.21 | 12.07,20.96 AREF.1
N$78
  Bottom 0.305: U8.10 24.98,26.04 C17.2 25.82,26.04 Q1.1
PB0
  Top 0.305: J25.30 5.71,47.62 6.99,46.35 10.16,46.35 20.32,36.2 U8.14
PB1  (via drill 0.6 pad 0.61)
  Top 0.305: U8.15 v9.53,36.2
  Bottom 0.305: J25.32 5.71,50.16 6.99,48.89 8.89,48.89 9.53,48.26 v9.53,36.2
PB2  (via drill 0.6 pad 0.61)
  Top 0.305: v10.16,34.29 12.07,34.29 12.7,33.66 U8.16
  Bottom 0.305: J25.34 5.71,52.7 6.99,51.43 9.53,51.43 10.16,50.8 10.16,37.46 10.8,36.83 10.8,35.56 10.16,34.92 v10.16,34.29
PB3/MOSI  (via drill 0.6 pad 0.61)
  Top 0.305: J23.4 34.29,3.17 30.48,3.17 24.13,9.53 24.13,15.88 22.86,17.15 20.32,17.15 17.78,19.69 17.78,23.5 15.88,25.4 v15.88,27.31 | v10.8,32.38 11.43,32.38 12.7,31.12 U8.17
  Bottom 0.305: J25.36 5.71,55.24 6.99,53.98 10.16,53.98 10.8,53.34 10.8,38.1 11.43,37.46 11.43,33.66 10.8,33.02 v10.8,32.38 | v15.88,27.31 15.88,30.48 15.24,31.12 U8.17
PB4/MISO
  Top 0.305: J23.1 36.2,8.89 29.21,8.89 27.3,10.79 27.3,17.15 23.49,20.96 23.49,21.59 22.86,22.23 19.68,22.23 19.05,22.86 19.05,26.67 17.14,28.58 U8.18
  Bottom 0.305: J25.38 5.71,57.78 6.99,56.52 9.53,56.52 11.43,54.61 11.43,38.73 12.07,38.1 12.07,29.21 12.7,28.58 U8.18
PB5/SCK  (via drill 0.6 pad 0.61)
  Top 0.305: J23.3 34.29,8.26 28.57,8.26 26.67,10.16 26.67,16.51 23.49,19.69 19.05,19.69 18.41,20.32 18.41,24.77 v17.14,26.04
  Bottom 0.305: J25.40 6.35,59.05 8.25,59.05 12.07,55.24 12.07,39.37 13.97,37.46 15.24,37.46 15.88,36.83 15.88,31.75 17.14,30.48 v17.14,26.04 U8.19
PC0  (via drill 0.6 pad 0.61)
  Top 0.305: v10.16,15.88 9.53,15.24 9.53,12.06 8.25,10.79 6.35,10.79 J25.2
  Bottom 0.305: v10.16,15.88 U8.23
PC1
  Bottom 0.305: J25.4 3.81,13.33 3.81,10.79 4.45,10.16 9.53,10.16 12.7,6.98 15.24,6.98 15.88,7.62 15.88,12.7 15.24,13.33 U8.24
PC2
  Bottom 0.305: U8.25 12.7,10.79 12.07,11.43 12.07,12.7 8.89,15.88 6.35,15.88 J25.6
PC3  (via drill 0.6 pad 0.61)
  Top 0.305: v6.35,13.33 6.35,18.42 J25.8
  Bottom 0.305: U8.26 12.7,8.26 11.43,9.53 11.43,11.43 9.53,13.33 v6.35,13.33
PC4  (via drill 0.6 pad 0.61)
  Top 0.305: U8.27 12.7,5.71 11.43,6.98 11.43,15.88 v8.89,18.42
  Bottom 0.305: v8.89,18.42 6.99,18.42 6.35,19.05 6.35,20.96 J25.10
PC5  (via drill 0.6 pad 0.61)
  Top 0.305: U8.28 12.7,3.17 12.07,3.81 12.07,5.08 8.25,8.89 5.71,8.89 3.81,10.79 v3.81,15.88
  Bottom 0.305: v3.81,15.88 3.81,23.5 J25.12
PC6/!RESET!
  Top 0.305: U8.1 D1.A
  Bottom 0.305: J23.5 25.53,6.98 R31.1 D1.A
PD0/RX  (via drill 0.6)
  Top 0.305: J25.14 5.71,27.31 6.99,26.04 8.25,26.04 8.89,25.4 8.89,19.69 12.07,16.51 12.07,15.24 12.7,14.61 15.24,14.61 16.51,13.33 16.51,9.53 20.32,5.71 U8.2 25.4,5.71 29.21,1.91 35.56,1.91 36.2,2.54 39.37,2.54 41.27,4.45 41.27,14.61 42.55,15.88 53.98,15.88 v54.61,15.24
  Bottom 0.305: v54.61,15.24 55.24,15.88 58.42,15.88 60.32,17.78 62.87,17.78 63.5,17.15 J64.1
PD1/TX
  Top 0.305: J25.16 5.71,29.85 6.99,28.58 8.25,28.58 9.53,27.31 9.53,20.32 12.7,17.15 15.24,17.15 15.88,16.51 15.88,15.24 17.14,13.97 17.14,11.43 20.32,8.26 U8.3 24.13,8.26 29.84,2.54 34.92,2.54 35.56,3.17 38.73,3.17 40.64,5.08 40.64,15.24 41.91,16.51 55.88,16.51 56.52,15.88 J64.2
PD2
  Top 0.305: J25.18 5.71,32.38 6.99,31.12 8.25,31.12 10.16,29.21 10.16,20.96 10.8,20.32 11.43,20.32 12.07,19.69 15.24,19.69 15.88,19.05 15.88,17.78 16.51,17.15 16.51,15.88 17.78,14.61 17.78,13.33 20.32,10.79 U8.4
PD3
  Top 0.305: J25.20 5.71,34.92 6.99,33.66 8.25,33.66 8.89,33.02 8.89,31.75 10.8,29.85 10.8,24.13 12.7,22.23 15.24,22.23 16.51,20.96 16.51,18.42 17.14,17.78 17.14,17.15 20.95,13.33 U8.5
PD4
  Top 0.305: J25.22 5.71,37.46 6.99,36.2 8.25,36.2 8.89,35.56 8.89,34.29 9.53,33.66 9.53,32.38 11.43,30.48 11.43,26.04 12.7,24.77 15.24,24.77 17.14,22.86 17.14,19.05 20.32,15.88 U8.6
PD5
  Top 0.305: J25.24 5.71,40 6.99,38.73 13.97,38.73 16.51,36.2 16.51,32.38 20.32,28.58 U8.11
PD6
  Top 0.305: J25.26 5.71,42.54 6.99,41.27 12.7,41.27 17.78,36.2 17.78,33.66 20.32,31.12 U8.12
PD7
  Top 0.305: J25.28 5.71,45.09 6.99,43.81 11.43,43.81 19.05,36.2 19.05,34.92 20.32,33.66 U8.13
RELAY_1
  Bottom 0.305: U12.1 85.09,45.09 85.09,43.81 83.82,42.54 83.82,41.27 82.55,40 82.55,38.73 81.28,37.46 81.28,36.2 78.74,33.66 78.74,29.85 72.39,23.5 J4.1
RELAY_2
  Bottom 0.305: U12.2 85.09,42.54 85.09,41.27 83.82,40 83.82,38.73 82.55,37.46 82.55,36.2 80.01,33.66 80.01,28.58 74.93,23.5 J4.2
RELAY_3
  Bottom 0.305: U12.3 85.09,40 85.09,38.73 83.82,37.46 83.82,36.2 81.28,33.66 81.28,27.31 77.47,23.5 J4.3
RELAY_4
  Bottom 0.305: J4.4 80.01,23.5 82.55,26.04 82.55,33.66 85.09,36.2 85.09,37.46 U12.4
RELAY_5
  Bottom 0.305: U12.5 83.82,33.66 83.82,24.77 82.55,23.5 J4.5
RELAY_6
  Bottom 0.305: J4.6 85.09,33.66 86.36,34.92 U12.6
RELAY_PWR
  Top 0.61: 97.79,28.58 J16.1 | J17.1 99.06,23.5 97.79,24.77 97.79,27.31 | 97.79,27.31 97.79,28.58 | U12.10 97.79,27.31 | J15.1 97.79,33.66 | 97.79,33.66 97.79,28.58 | J14.1 97.79,38.73 | 97.79,38.73 97.79,33.66 | J13.1 97.79,43.81 | 97.79,43.81 97.79,38.73 | J12.1 97.79,48.89 | 97.79,48.89 97.79,43.81 | J6.1 99.06,55.24 97.79,53.98 97.79,48.89
RLY1
  Bottom 0.61: U12.18 95.89,47.62 99.7,51.43 J12.2
RLY2
  Bottom 0.61: U12.17 96.52,45.09 97.79,46.35 J13.2
RLY3
  Bottom 0.61: U12.16 96.52,42.54 97.79,41.27 J14.2
RLY4
  Bottom 0.61: U12.15 96.52,40 97.79,38.73 97.79,37.46 99.06,36.2 J15.2
RLY5
  Bottom 0.61: U12.14 95.89,37.46 97.79,35.56 97.79,33.02 99.7,31.12 J16.2
RLY6
  Bottom 0.61: U12.13 93.98,34.92 92.71,33.66 92.71,27.31 93.98,26.04 J17.2
SCLK  (via drill 0.6 pad 0.61)
  Top 0.305: U6.7 16.51,60.96 17.78,59.69 17.78,56.52 20.32,53.98 20.32,50.8 19.05,49.53 U10.3 | J11.1 66.04,17.78 62.23,21.59 v62.23,22.86
  Bottom 0.305: v62.23,22.86 62.23,24.13 64.14,26.04 64.77,26.04 66.68,27.94 66.68,28.58 64.14,31.12 40.64,31.12 39.37,32.38 39.37,36.2 38.73,36.83 24.77,36.83 19.05,42.54 U10.3
V+
  Top 0.5: J1.1 81.92,6.98 85.73,10.79 85.73,19.69 88.27,22.23 J7.3

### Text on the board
Top: SENSE
tTest: 1 | 2 | 3 | 4 | 5 | 6 | 7 | 8 | 9 | 10 | 11 | 12 | AD1 | AD0 | A | DA1 | B | DA0 | PWR | PB5 | PB4 | PB3 | PWR | PB2 | 1 | PB1 | PB0 | 2 | PD7 | PD6 | 3 | PD5 | Bertboard | 10/2012 | PD4 | 4 | PD3 | GND | PD2 | 5 | PD1 | MOTOR | XTAL | A | B | PD0 | 6 | 1 | 2 | 3 | 4 | 5 | 6 | PC5 | PC4 | 1 | 2 | 3 | 4 | PC3 | RELAY | V_SRC | C2 | GP4 | GP1 | GP0 | 3V3 | C1 | C0 | 25 | 24 | 9 | 8 | 7 | 4 | 1 | 0 | 5V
